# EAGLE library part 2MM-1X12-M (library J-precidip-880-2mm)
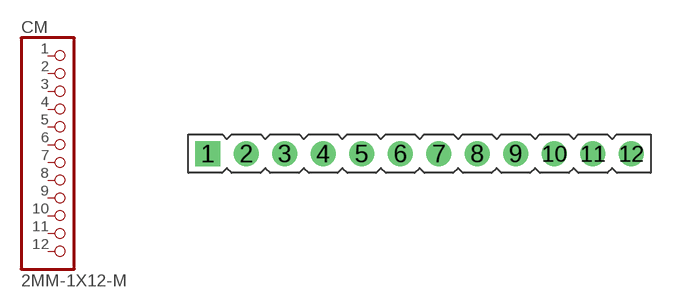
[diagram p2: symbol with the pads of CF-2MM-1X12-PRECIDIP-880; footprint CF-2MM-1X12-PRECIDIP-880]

Designator prefix CM

## 2MM-1X12-M  [CF-2MM-1X12-PRECIDIP-880]
1  1  pas
2  2  pas
3  3  pas
4  4  pas
5  5  pas
6  6  pas
7  7  pas
8  8  pas
9  9  pas
10  10  pas
11  11  pas
12  12  pas

## Footprint CF-2MM-1X12-PRECIDIP-880 (pad centres in mm)
drill 0.8 square: 1 -11,0
drill 0.8: 2 -9,0; 3 -7,0; 4 -5,0; 5 -3,0; 6 -1,0; 7 1,0; 8 3,0; 9 5,0; 10 7,0; 11 9,0; 12 11,0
